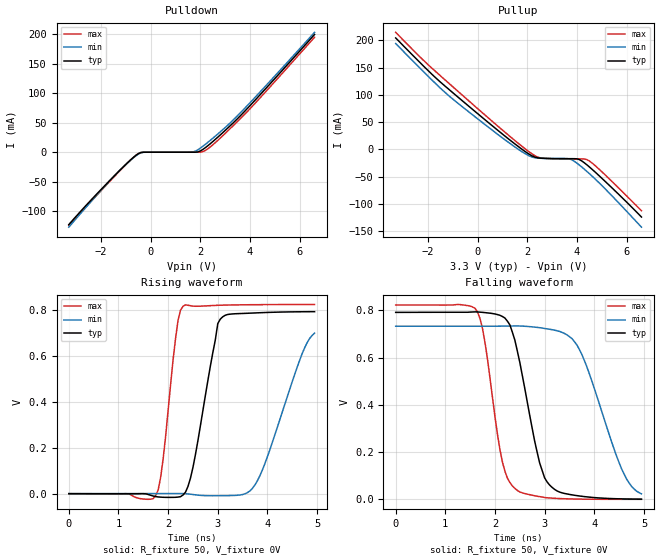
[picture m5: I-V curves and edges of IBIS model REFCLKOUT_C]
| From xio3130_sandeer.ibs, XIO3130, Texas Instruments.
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[Model] REFCLKOUT_C
Model_type Output
Polarity Non-Inverting
Cref = 2.0pF
Rref = 50
Vref = 0V
Vmeas =0.350V
| typ min max
C_comp   2.0pF   1.5pF   3.0pF
|Voh = 0.42V
|Vol = 0.105V
|[Model Spec]
| typ min max
|   typ   min   max
|Voh   1.1V   0.42V   1.61V
|Vol   0.01V   -0.3V   0.105V
[Temperature Range]   25   125   -40
[Voltage Range] 3.30V 3.00V 3.60V
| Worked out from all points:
|   slope of the pullup table from 0 to 0.495 V, typ, clamps not added: 26.5 ohm
|   rising waveform, R_fixture 50, V_fixture 0V: 20-80 % time 379ps typ, 649ps min, 234ps max; typ from 0.001 V to 0.791 V
|   falling waveform, R_fixture 50, V_fixture 0V: 20-80 % time 450ps typ, 688ps min, 341ps max; typ from 0.791 V to 0.001 V
| (Vdd votage range) 1.50V 1.35V 1.65V
| (Process strength) nominal weak strong
[Pulldown]
-3.3V     -122.7mA   -127.1mA   -124.1mA
-1.5V     -41.47mA   -41.63mA   -42.75mA
-900mV    -16.46mA   -16.86mA   -16.77mA
-500mV    -2.49mA    -3.215mA   -2.209mA
-300mV    -33.12uA   -144.9uA   -12.3uA
1.7V      1.372uA    437.4uA    4.038nA
2V        2.19mA     7.016mA    112.8uA
2.3V      11.03mA    16.77mA    5.763mA
3V        37.03mA    41.93mA    31.95mA
3.6V      61.41mA    66.37mA    56.62mA
4.6V      106.5mA    111.1mA    101.2mA
6.6V      199.8mA    203.4mA    195.1mA
[Pullup]
-3.3V     204.1mA    193.9mA    214.4mA
-2.2V     153.6mA    143.3mA    164mA
-1.1V     107.8mA    96.05mA    118.8mA
1.1V      24.6mA     17.86mA    31.67mA
2.1V      -9.254mA   -12.08mA   -5.117mA
2.6V      -16.04mA   -16.19mA   -15.68mA
3.6V      -16.82mA   -16.6mA    -17.15mA
3.9V      -16.85mA   -21.74mA   -17.19mA
4.1V      -18.48mA   -28.52mA   -17.2mA
4.3V      -24.38mA   -36.08mA   -17.34mA
4.6V      -35.83mA   -48.24mA   -24.35mA
6.6V      -123.6mA   -142.1mA   -112mA
[Ramp]
| variable   typ   min   max
dV/dt_r 0.474231V/0.378831ns  0.439211V/0.684942ns  0.493192V/0.23448ns
dV/dt_f 0.474264V/0.450396ns  0.438984V/0.713104ns  0.493432V/0.340973ns
R_load = 50
[Rising Waveform]
R_fixture = 50
V_fixture = 0V
V_fixture_min = 0V
V_fixture_max = 0V
0s        615.1uV    981.7uV    12.96uV
1.75ns    -12.14mV   981.7uV    -7.037mV
1.9ns     -15.12mV   981.7uV    151.8mV
2.2ns     -14.21mV   1.036mV    753.7mV
2.3ns     -5.309mV   871.5uV    814mV
2.5ns     114.3mV    -3.158mV   815mV
3ns       738.9mV    -8.365mV   818.6mV
3.6ns     783.9mV    5.298mV    820.8mV
3.9ns     786.7mV    104.5mV    821.4mV
4.95ns    790.9mV    697.8mV    822mV
|   5E-09S   0.791V   0.7042V   0.822
|   5.05E-09S   0.791V   0.7092V   0.822
|   5.1E-09S   0.791V   0.7124V   0.822
|   5.15E-09S   0.791V   0.7151V   0.822
|   5.2E-09S   0.791V   0.7171V   0.822
|   5.25E-09S   0.791V   0.7188V   0.822
|   5.3E-09S   0.791V   0.7201V   0.822
|   5.35E-09S   0.791V   0.7213V   0.822
|   5.4E-09S   0.791V   0.7223V   0.822
|   5.45E-09S   0.791V   0.7232V   0.822
|   5.5E-09S   0.791V   0.724V   0.822
|   5.55E-09S   0.791V   0.7247V   0.822
|   5.6E-09S   0.791V   0.7254V   0.822
|   5.65E-09S   0.791V   0.726V   0.822
|   5.7E-09S   0.791V   0.7265V   0.822
|   5.75E-09S   0.791V   0.727V   0.822
|   5.8E-09S   0.791V   0.7275V   0.822
|   5.85E-09S   0.791V   0.728V   0.822
|   5.9E-09S   0.791V   0.7284V   0.822
|   5.95E-09S   0.791V   0.7288V   0.822
|   6E-09S   0.791V   0.7292V   0.822
|   6.05E-09S   0.791V   0.7295V   0.822
|   6.1E-09S   0.791V   0.7298V   0.822
|   6.15E-09S   0.791V   0.7302V   0.822
|   6.2E-09S   0.791V   0.7304V   0.822
|   6.25E-09S   0.791V   0.7307V   0.822
|   6.3E-09S   0.791V   0.731V   0.822
|   6.35E-09S   0.791V   0.7312V   0.822
|   6.4E-09S   0.791V   0.7314V   0.822
|   6.45E-09S   0.791V   0.7316V   0.822
|   6.5E-09S   0.791V   0.7317V   0.822
|   6.55E-09S   0.791V   0.7319V   0.822
|   6.6E-09S   0.791V   0.7321V   0.822
|   6.65E-09S   0.791V   0.7322V   0.822
|   6.7E-09S   0.791V   0.7323V   0.822
|   6.75E-09S   0.791V   0.7325V   0.822
|   6.8E-09S   0.791V   0.7326V   0.822
|   6.85E-09S   0.791V   0.7327V   0.822
|   6.9E-09S   0.791V   0.7328V   0.822
|   6.95E-09S   0.791V   0.7329V   0.822
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[Falling Waveform]
R_fixture = 50
V_fixture = 0V
V_fixture_min = 0V
V_fixture_max = 0V
0s        791.1mV    732.6mV    822.4mV
1.6ns     793.3mV    732.6mV    807.8mV
1.75ns    791.2mV    732.6mV    720.9mV
2.2ns     767.3mV    732.9mV    118.9mV
2.4ns     673.9mV    733.7mV    46.57mV
3ns       90.69mV    722.9mV    7.627mV
3.45ns    22.79mV    696.1mV    2.149mV
3.8ns     11.58mV    587.4mV    722.1uV
4.55ns    1.959mV    129mV      71.02uV
4.95ns    748.5uV    23.16mV    17.81uV
